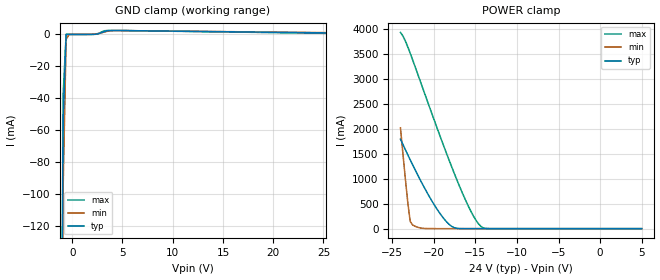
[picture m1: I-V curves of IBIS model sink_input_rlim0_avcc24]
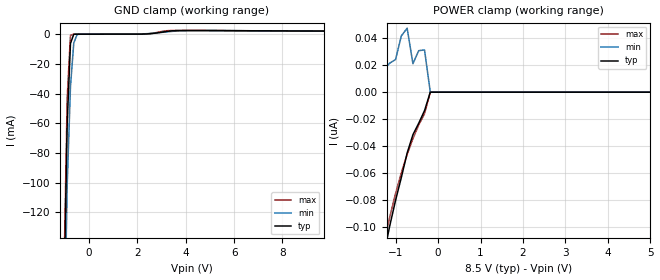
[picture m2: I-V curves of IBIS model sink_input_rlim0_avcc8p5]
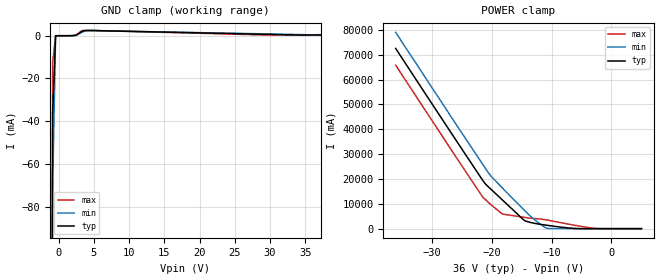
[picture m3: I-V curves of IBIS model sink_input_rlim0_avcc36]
| IBIS file created by Layout Workbench Version 22.1.4.12161.401368   004
| Cadence Design Systems, Inc. 2011
| Texas Instruments Incorporated
| ISO1228 Eight-Channel Isolated 24-V Digital Input Receivers
[IBIS ver] 4.2
[File name]  iso1228.ibs
[File Rev]  1.0
[Date]   01 29, 2024
[Source]
| Texas Instruments Incorporated.
| 12500 TI Blvd
| Dallas, TX -75243
[Notes]   Revision History:
|   Rev 1.0: 01/30/2024
| - Initial version of the model
| - Field side model is provided only for sinking type inputs
| - Model generated from Cadence T2B tool
| - C_comp although listed in numerical order of value are
|   obtained from varying PVT conditions. For PVT conditions for
|   each specific value refer the buffer description under
|   respective [Model]. IBIS model user is responsible for using
|   appropriate C_comp to simulate for Signal Integrity.
| - Warnings regarding combined Non-monotonicity of various models have been
|   reviewed and considered minor and can be ignored.
| - Model names with a trailing _3p3 contain the model for 3.3V operation.
|   Model names with a trailing _5p0 contain the model for 5.0V operation.
| - Pins with model_name as inout behave as input when COMM_SEL=1, and output when COMM_SEL=0
| - Pin 31 (OUT5_nINT) can be either output(COMM_SEL=0) or open drain(COMM_SEL=1) depending upon state of COMM_SEL.
|   The model is for output which covers both the cases
[Disclaimer]
| This model is designed as an aid for customers of Texas Instruments.
| TI and its licensors and suppliers make no warranties, either expressed
| or implied, with respect to this  model, including the warranties of
| merchantability or fitness for a particular purpose. The model is
| provided solely on an "as is" basis. The entire risk as to its quality
| and performance is with the customer.
| This model is subject to change without notice. Texas Instruments
| Incorporated is not responsible for updating this model
[Copyright]
(C) Copyright 2024 Texas Instruments Incorporated.All rights reserved.
|   Component ISO1228
[Component] ISO1228
[Manufacturer] TI
[Package] |38 DFB
| variable   typ   min   max
R_pkg   0.52   0.52   0.52
L_pkg   5.2nH   5.2nH   5.2nH
C_pkg   1.04nF   1.04nF   1.04nF
[Pin]  signal_name   model_name   R_pin   L_pin   C_pin
1   IN1   input
2   LED1   Gnd
3   IN2   input
4   LED2   Gnd
5   IN3   input
6   LED3   Gnd
7   AVSS   Gnd
8   IN4   input
9   LED4   Gnd
10   IN5   input
11   LED5   Gnd
12   IN6   input
13   LED6   Gnd
14   IN7   input
15   LED7   Gnd
16   AVCC   Power
17   AVSS   Gnd
18   IN8   input
19   LED8   Gnd
20   NC   NC
21   GND1   Gnd
22   NC   NC
23   F1   trilvl
24   F0   trilvl
25   GND1   Gnd
26   nFAULT   opendrain
27   OUT_EN   out_en
28   OUT8_SYNC   output
29   OUT7_BURSTEN   inout
30   OUT6_nRST   inout
31   OUT5_nINT   output
32   OUT4_nCS   inout
33   OUT3_SCLK   inout
34   OUT2_SDI   inout
35   OUT1_SDO   output
36   GND1   Gnd
37   VCC1   Power
38   COMM_SEL   comm_sel
[Model Selector] input
sink_input_rlim0_avcc24 0ohm 24V
sink_input_rlim0_avcc8p5 0ohm 8.5V
sink_input_rlim0_avcc36 0ohm 36V
sink_input_rlim1k_avcc24 1kohm 24V
sink_input_rlim1k_avcc8p5 1kohm 8.5V
sink_input_rlim1k_avcc36 1kohm 36V
[Model Selector] output
output_3p3  3.3V VCC1 Digital Output
output_5p0  5.0V VCC1 Digital Output
[Model Selector] trilvl
trilvl_3p3  3.3V VCC1 Tri-level Input
trilvl_5p0  5.0V VCC1 Tri-level Input
[Model Selector] inout
inout_3p3   3.3V VCC1 Digital I/O
inout_5p0   5.0V VCC1 Digital I/O
[Model Selector] comm_sel
comm_sel_3p3  3.3V VCC1 Input
comm_sel_5p0  5.0V VCC1 Input
[Model Selector] opendrain
opendrain_3p3  3.3V VCC1 OD output
opendrain_5p0  5.0V VCC1 OD output
| Models and submodels in the file (17): sink_input_rlim0_avcc24 (Input), sink_input_rlim0_avcc8p5 (Input), sink_input_rlim0_avcc36 (Input), sink_input_rlim1k_avcc24 (Input), sink_input_rlim1k_avcc8p5 (Input), sink_input_rlim1k_avcc36 (Input), comm_sel_3p3 (Input), comm_sel_5p0 (Input), output_3p3 (Output), output_5p0 (Output), inout_3p3 (I/O), inout_5p0 (I/O), out_en (Input), trilvl_3p3 (Input), trilvl_5p0 (Input), opendrain_3p3 (Open_drain), opendrain_5p0 (Open_drain)
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|   Model sink_input_rlim0_avcc24
[Model] sink_input_rlim0_avcc24
Model_type Input
Vinl =  5.100V
Vinh =  6.000V
C_comp   0.859pF   0.874pF   1.06pF
[Model Spec]
Vinh   6.000V   5.700V   6.400V
Vinl   5.100V   4.700V   5.300V
[Temperature Range]   27.000   0.150k   -40.000
[Voltage Range]   24.000V   24.000V   24.000V
[GND_clamp]
|Voltage   I(typ)   I(min)   I(max)
-24V      -39.17A    -38.93A    -39.33A
-1.192V   -364.9mA   -400.2mA   -356.7mA
-899mV    -54.96mA   -94.74mA   -37.62mA
-606mV    -31.67uA   -3.096mA   -1.238uA
-313mV    -342.2nA   -2.054uA   -415.5nA
2.323V    104.3uA    260.1uA    82.32uA
3.202V    1.796mA    1.492mA    2.306mA
4.374V    2.453mA    2.394mA    2.484mA
48V       -686.1uA   -332.6uA   -1.295mA
[POWER_clamp]
|Voltage   I(typ)   I(min)   I(max)
-24V      1.793A     2.021A     3.931A
-23.12V   1.481A     526.4mA    3.642A
-22.83V   1.379A     143.6mA    3.514A
-22.54V   1.279A     72.45mA    3.381A
-19.9V    467.3mA    606uA      2.154A
-18.14V   85mA       358.3uA    1.367A
-17.26V   8.109mA    276.4uA    996.1mA
-15.8V    538.8uA    142uA      437.8mA
-14.92V   440.7uA    76.24uA    167.9mA
-14.33V   378.8uA    34.12uA    45.58mA
-13.46V   286.4uA    -1.503uA   1.43mA
5V        0A         0A         0A
|   Model sink_input_rlim0_avcc8p5
[Model] sink_input_rlim0_avcc8p5
Model_type Input
Vinl =  5.100V
Vinh =  6.000V
C_comp   0.859pF   0.874pF   1.06pF
[Model Spec]
Vinh   6.000V   5.700V   6.400V
Vinl   5.100V   4.700V   5.300V
[Temperature Range]   27.000   0.150k   -40.000
[Voltage Range]   8.500V   8.500V   8.500V
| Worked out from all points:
|   GND clamp passes 1 mA (typ) near -0.66 V on its own axis
[GND_clamp]
|Voltage   I(typ)   I(min)   I(max)
-8.5V     -12.68A    -12.59A    -12.74A
-1.045V   -181mA     -225.2mA   -164.1mA
-909mV    -60.32mA   -101.7mA   -42.74mA
-773mV    -6.233mA   -35.31mA   -784.2uA
-636mV    -84.79uA   -5.912mA   -2.411uA
-500mV    -1.06uA    -254.1uA   -728.8nA
2.364V    132.2uA    294.9uA    113.4uA
3.182V    1.748mA    1.459mA    2.277mA
3.864V    2.418mA    2.32mA     2.492mA
17V       1.555mA    1.636mA    1.398mA
[POWER_clamp]
|Voltage   I(typ)   I(min)   I(max)
-8.5V     -3.676uA   -2.622uA   -4.119uA
-2.5V     -381.9nA   -106.7nA   -372.1nA
-1.818V   -219.6nA   -19.81nA   -207.3nA
-1.273V   -119.3nA   17.01nA    -111.4nA
-1.136V   -98.73nA   21.48nA    -92.18nA
-1V       -79.98nA   24.15nA    -74.95nA
-864mV    -63.05nA   41.62nA    -59.59nA
-727mV    -44.95nA   47.3nA     -46.05nA
-591mV    -31.45nA   21.04nA    -34.34nA
-318mV    -13.65nA   31.25nA    -15.94nA
-182mV    0A         0A         0A
5V        0A         0A         0A
|   Model sink_input_rlim0_avcc36
[Model] sink_input_rlim0_avcc36
Model_type Input
Vinl =  5.100V
Vinh =  6.000V
C_comp   0.859pF   0.874pF   1.06pF
[Model Spec]
Vinh   6.000V   5.700V   6.400V
Vinl   5.100V   4.700V   5.300V
[Temperature Range]   27.000   0.150k   -40.000
[Voltage Range]   36.000V   36.000V   36.000V
[GND_clamp]
|Voltage   I(typ)   I(min)   I(max)
-36V      -59.67A    -59.3A     -59.9A
-1.273V   -477.6mA   -508mA     -473.9mA
-859mV    -36.13mA   -70.22mA   -12.46mA
-444mV    -569.5nA   -59.19uA   -630.1nA
2.04V     18.99uA    92.16uA    12.28uA
2.455V    216.4uA    384.2uA    222.5uA
3.283V    1.977mA    1.627mA    2.38mA
3.697V    2.392mA    2.207mA    2.476mA
4.939V    2.431mA    2.407mA    2.447mA
29.79V    627.2uA    821.5uA    316.3uA
34.34V    310.6uA    530.2uA    376.9uA
72V       661.2uA    -1.853mA   2.008mA
[POWER_clamp]
|Voltage   I(typ)   I(min)   I(max)
-36V      72.54A     79A        65.79A
-21.5V    19.55A     25.97A     12.83A
-21.09V   18.14A     24.49A     11.84A
-20.26V   16.22A     21.61A     9.992A
-18.19V   11.53A     16.36A     5.913A
-14.46V   3.172A     7.236A     4.531A
-12.39V   1.947A     2.745A     4A
-10.74V   1.347A     98.54mA    3.471A
-6.182V   90.39mA    361.9uA    1.383A
-2.869V   13.24uA    74.11uA    153.8mA
5V        0A         0A         0A
